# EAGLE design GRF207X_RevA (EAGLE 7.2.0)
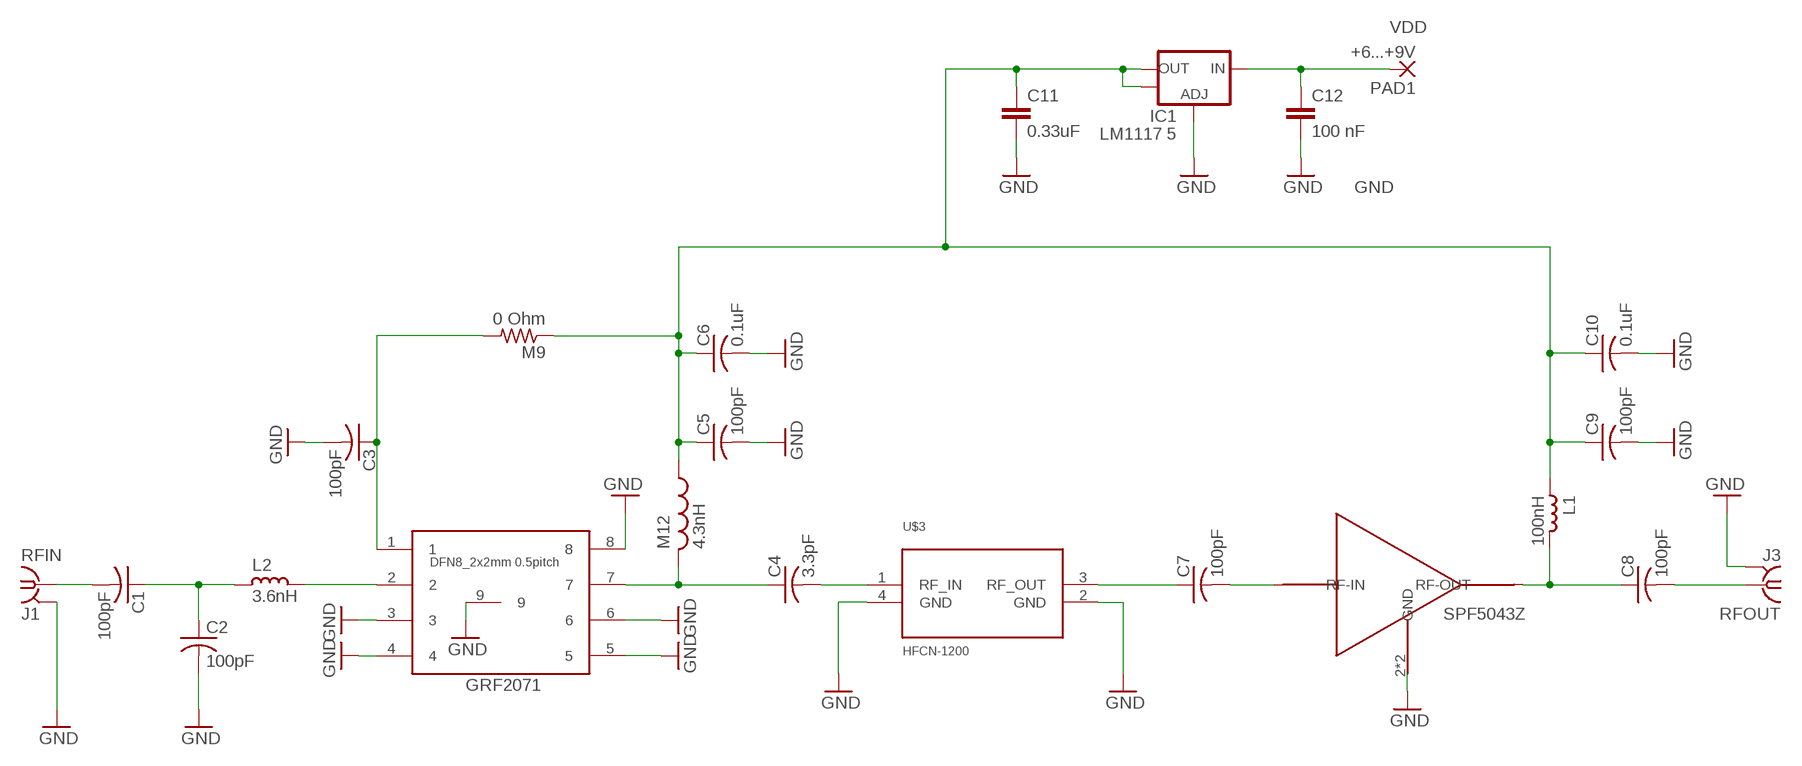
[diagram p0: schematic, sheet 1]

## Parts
C1  100pF  RCL_C0402_GRF30WIDE  [RCL_C-US_GRF_30WIDE]
C2  100pF  RCL_C0402_GRF30WIDE  [RCL_C-US_GRF_30WIDE]
C3  100pF  RCL_C0402_GRFWIDE  [RCL_C-US_GRF_NARROW]
C4  3.3pF  RCL_C0402_GRF30WIDE  [RCL_C-US_GRF_30WIDE]
C5  100pF  C-USC0603  [C0603]
C6  0.1uF  RCL_C0402_GRF30WIDE  [RCL_C-US_GRF_30WIDE]
C7  100pF  C-USC0603  [C0603]
C8  100pF  C-USC0603  [C0603]
C9  100pF  C-USC0603  [C0603]
C10  0.1uF  C-USC0603  [C0603]
C11  0.33uF  C-EUC0805  [C0805]
C12  100 nF  C-EUC0805  [C0805]
IC1  LM1117 5  V_REG_LM1117SOT223  [SOT223]
L1  100nH  L_0603  [L0603]
L2  3.6nH  L_0603  [L0603]
M9  0 Ohm  R-US_R0402  [R0402]
M12  4.3nH  L-US_L0402_WIDENORMAL  [RCL_L-US_L0402]
PAD1  +6...+9V  WIREPAD1,6/0,8  [1,6/0,8]
RFIN  J1  SMA-142-0701-801/806  [J502-ND-142-0701-801/806]
RFOUT  J3  SMA-142-0701-801/806  [J502-ND-142-0701-801/806]
SPF5043Z  SPF5043Z  PSA4-5043+  [PSA4-5043+]
U1  DFN8_2X2MM  [DFN8_2X2MM]
U$3  HFCN-1200  [HFCN-1200]

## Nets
GND: C2.2 C3.2 C5.2 C6.2 C9.2 C10.2 C11.2 C12.2 IC1.1(ADJ) RFIN.G@1 RFIN.G@2 RFIN.G@3 RFIN.G@4 RFOUT.G@1 RFOUT.G@2 RFOUT.G@3 RFOUT.G@4 SPF5043Z.2(GND) SPF5043Z.4(GND) U1.3 U1.4 U1.5 U1.6 U1.8 U1.9 U$3.2(GND) U$3.4(GND)
N$1 [RFIN]: C1.2 RFIN.1
N$2 [POWER]: C5.1 C6.1 C9.1 C10.1 C11.1 IC1.2(OUT) IC1.4(OUT) L1.2 M9.1 M12.1
N$3 [RFOUT]: C4.2 U$3.1(RF_IN)
N$4 [RFIN]: L2.1 U1.2
N$5 [RFOUT]: C7.1 U$3.3(RF_OUT)
N$6 [RFIN]: C1.1 C2.1 L2.2
N$7 [RFOUT]: C4.1 M12.2 U1.7
N$8 [RFOUT]: C7.2 SPF5043Z.3(RF-IN)
N$9 [RFOUT]: C8.1 L1.1 SPF5043Z.1(RF-OUT)
N$10 [RFOUT]: C8.2 RFOUT.1
N$11 [POWER]: C12.1 IC1.3(IN) PAD1.1(P)
VRX [POWER]: C3.1 M9.2 U1.1

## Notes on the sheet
- VDD
- GND
- SPF5043Z
- GRF2071

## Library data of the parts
C1-C4 C6 = GuerrillaRF:RCL_C0402_GRF
C5 C7-C10 = adafruit:C-US: CAPACITOR, American symbol
C11 C12 = resistor:C-EU: CAPACITOR, European symbol
IC1 = SparkFun-PowerIC:V_REG_LM1117: Voltage Regulator LM1117 Standard adjustable voltage regulator but in SMD form. Spark Fun Electronics SKU : COM-00595
L1 L2 = rc-master-smd:L_: INDUCTOR
M9 = rcl:R-US_: RESISTOR, American symbol
M12 = GuerrillaRF:L-US_L0402_WIDE
PAD1 = wirepad:WIREPAD: Wire PAD connect wire on PCB
RFIN RFOUT = GuerrillaRF:SMA-: SMA 50 Ohm End Launch Jack Receptacle - Round Contact; MF: JOHNSON COMPONENTS; MPN: 142-0701-801; OC_FARNELL: 1608592; OC_NEWARK: 90F2624
SPF5043Z = Ava:PSA4-5043+
U1 = GuerrillaRF:DFN8_2X2MM
U$3 = HFCN-1200:HFCN-1200: HFCN-1200+ HFCN-1200 High Pass Filter

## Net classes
0 default: drill 0.152 mm, clearance 0.152 mm
1 RFIN: clearance 0.508 mm to class 0
2 RFOUT: clearance 0.508 mm to class 0
3 POWER: clearance 0.254 mm to class 0
4 FID: clearance 0.178 mm to class 0
5 NC: clearance 0.178 mm to class 0
6 Bypass: clearance 0.203 mm to class 0

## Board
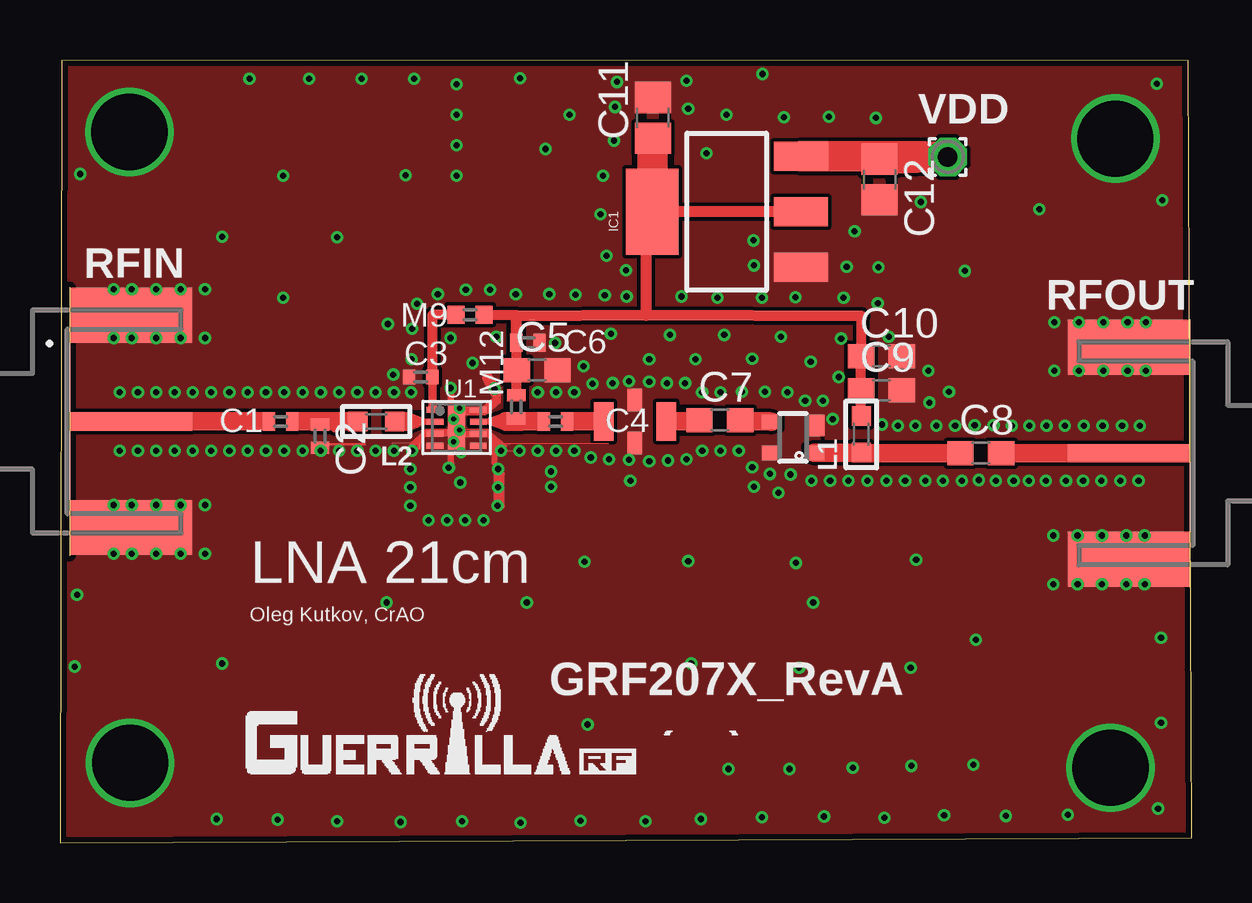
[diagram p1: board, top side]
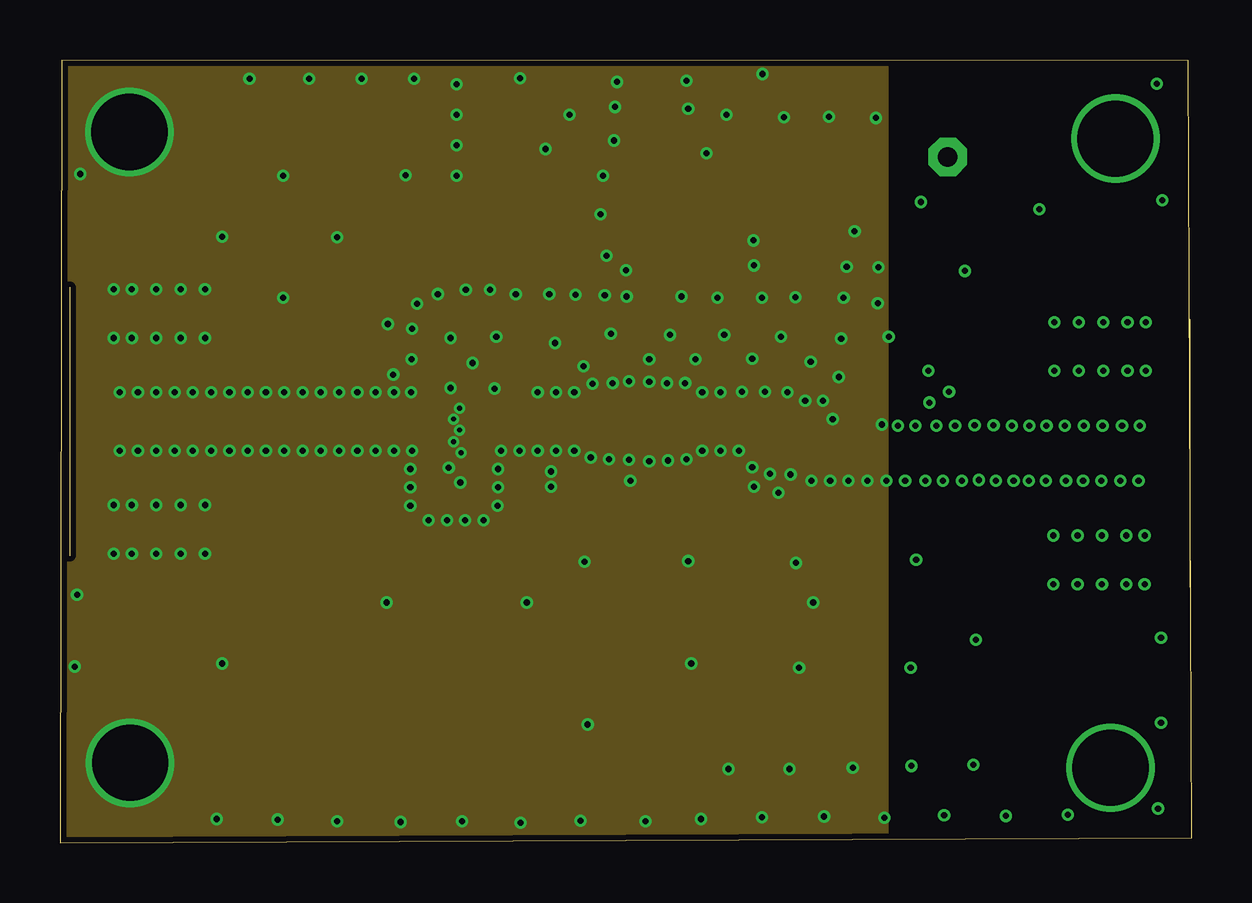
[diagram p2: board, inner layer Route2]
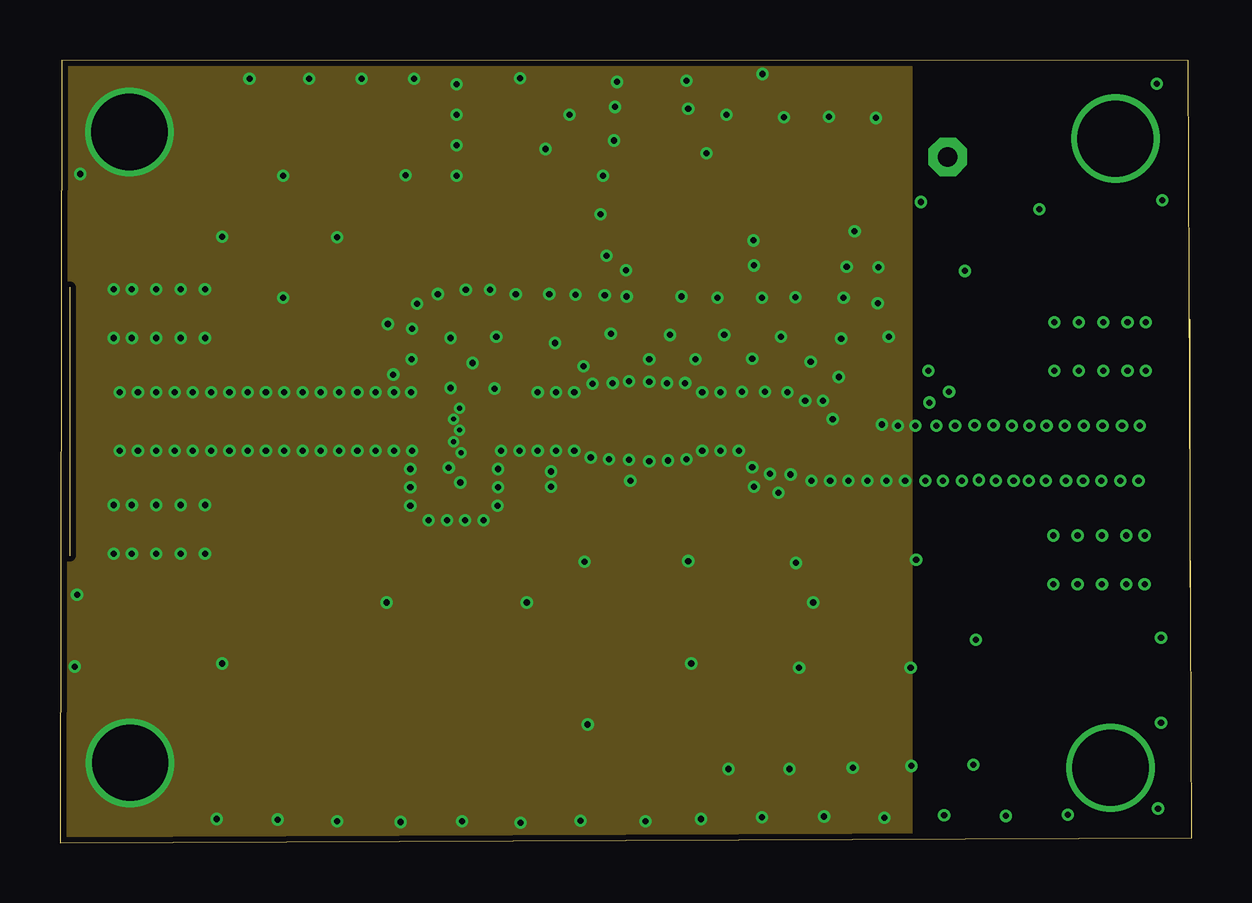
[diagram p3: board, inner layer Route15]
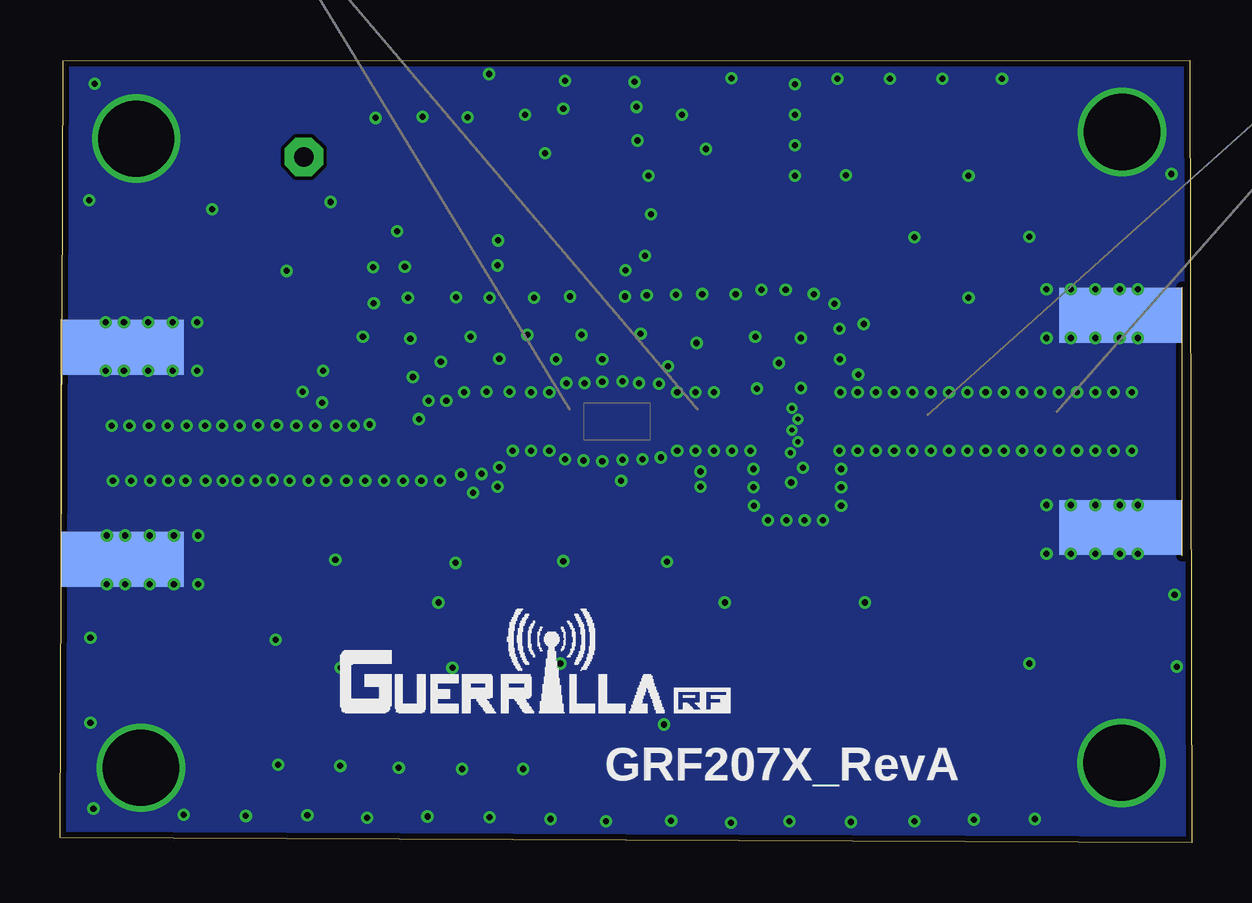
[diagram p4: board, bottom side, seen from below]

Size 47.17 x 32.61 mm. Coordinates in mm from the lower left corner, seen from the top.
Outline: 0,0 47.17,0.2 47.04,32.59 0.08,32.61 0,0
Copper layers (1*2*15*16): Top 0.035559375mm / dielectric 16mil / Route2 0.035559375mm / dielectric 24mil / Route15 0.035559375mm / dielectric 16mil / Bottom 0.035559375mm
Design rules "Eugene_Design_Rules_rev2": minimum track width 1mil, minimum drill 8mil, track to track 6mil, track to pad 4mil, pad to pad 4mil, via to via 4mil, smd to smd 0mil, copper to edge 10mil, drill to drill 8mil, minimum pad ring 5mil, minimum via ring 5mil, stop-mask expansion 0mil, vias tented up to drill 10mil, thermal gap 0mil

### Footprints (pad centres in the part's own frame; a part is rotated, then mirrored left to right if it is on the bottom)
RCL_C-US_GRF_30WIDE = smd 0.508 x 0.762: 1 -0.483,0; 2 0.483,0
RCL_C-US_GRF_NARROW = smd 0.508 x 0.61: 1 -0.483,0; 2 0.483,0
C0603 = smd 1.1 x 1: 1 -0.85,0; 2 0.85,0
C0805 = smd 1.3 x 1.5: 1 -0.85,0; 2 0.85,0
SOT223 = smd 1.219 x 2.235: 1 -2.311,-3.099; 2 0,-3.099; 3 2.311,-3.099 | smd 3.6 x 2.2: 4 0,3.099
L0603 = smd 0.8 x 0.8: 1 -0.762,0; 2 0.762,0
R0402 = smd 0.711 x 0.762: 1 -0.584,0; 2 0.584,0
RCL_L-US_L0402 = smd 0.508 x 0.762: 1 -0.483,0; 2 0.483,0
1,6/0,8 = drill 0.813 pad 1.6 octagon: 1 0,0
J502-ND-142-0701-801/806 = smd 5.08 x 0.762: 1 2.565,0 | smd 5.08 x 2.286: G@1 2.565,4.42; G@2 2.565,-4.42 | smd 5.08 x 2.286 bottom: G@3 2.565,4.42; G@4 2.565,-4.42
PSA4-5043+ = smd 0.6 x 0.8: 1 -0.65,-0.9; 3 0.65,0.9; 4 -0.65,0.9 | smd 0.9 x 0.8: 2 0.5,-0.9
DFN8_2X2MM = smd 0.7 x 0.25: 1 -0.9,0.75; 2 -0.9,0.25; 3 -0.9,-0.25; 4 -0.9,-0.75; 5 0.9,-0.75; 6 0.9,-0.25; 7 0.9,0.25; 8 0.9,0.75 | smd 0.7 x 1.8: 9 0,0
HFCN-1200 = smd 0.813 x 1.6: 1 -0.406,0; 3 2.21,0 | smd 0.61 x 0.94: 2 0.889,-0.889; 4 0.889,0.889

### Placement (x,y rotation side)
C1  9.19,17.55 180 top
C2  10.85,16.94 270 top
C3  15.04,19.41 180 top
C4  20.65,17.55 0 top
C5  19.89,19.69 0 top
C6  19.51,20.83 0 top
C7  27.51,17.6 0 top
C8  38.38,16.23 0 top
C9  34.24,18.85 0 top
C10  34.24,20.27 0 top
C11  24.71,30.2 90 top
C12  34.16,27.64 270 top
IC1  27.79,26.29 90 top
L1  33.4,17.02 90 top
L2  13.18,17.55 180 top
M9  17.09,22 180 top
M12  19.02,18.16 270 top
PAD1  37.01,28.58 0 top
RFIN  0.41,17.55 0 top
RFOUT  47.12,16.23 180 top
SPF5043Z  30.56,16.89 90 top
U1  16.54,17.3 0 top
U$3  23.06,17.55 0 top

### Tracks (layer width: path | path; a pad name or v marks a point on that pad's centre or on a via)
GND  (via drill 0.2, 0.25, 3.17)
  Top 0.051: 14.61,16.64 15.27,17.22 16.28,17.22 | 14.61,16.64 13.84,16.64 v13.92,16.33 | 14.61,16.64 14.73,16.64 14.66,16.51 | 15.44,17.07 15.65,17.04 | 15.65,17.04 16.54,16.92 v16.66,17.2 | 11,16.61 11.63,16.61 v11.63,16.33 | 21.44,16.64 22.86,16.64 | v21.44,16.33 21.44,16.64 | 18.21,15.6 18.16,15.6 18.26,15.39 | U1.3 15.65,17.04 | v16.21,15.62 16.31,15.8 | 14.99,16.41 14.73,16.38 v14.68,16.33 | 18.34,18.34 17.73,17.83 16.89,17.83 v16.66,18.11 | 18.36,18.95 18.34,18.34 | 16.87,17.22 17.81,17.22 18.49,16.64 18.82,16.64 | 18.82,16.64 21.44,16.64 | 16.89,16.92 17.83,16.92 | 17.83,16.92 18.52,16.33 19.41,16.33 | 17.68,18.01 U1.8 | 17.81,17.07 U1.6 | 17.83,17.04 U1.6 | 17.83,16.92 U1.6 | 18.49,16.51 18.82,16.64 | 18.11,15.85 v18.26,15.57 | 18.34,18.34 17.92,18.22 | 15.01,16.84 14.95,16.57
  Top 0.102: 11,16.61 12.7,16.61 | 15.01,16.84 14.99,16.41 | 15.09,16.87 14.95,16.57 14.88,16.43
  Top 0.254: 14.66,16.51 15.29,17.09 16.26,17.09 | 15.44,17.07 16.46,17.07 | 18.21,14.25 18.21,15.6 | 18.42,14.02 18.42,15.37 | 16.31,15.8 16.31,17.15 | 16.87,17.07 17.81,17.07 | 18.49,16.51 17.83,17.04 | 18.11,15.85 18.11,16.79 | 16.31,17.32 16.31,18.67
  Top 0.356: 16.87,18.01 17.68,18.01 | 17.68,18.01 17.7,18.01 | 17.68,18.01 17.92,18.22 18.19,18.44
  Top 0.457: 17.83,19.35 18.16,18.75
  other vias: 31.06,18.42 31.8,18.42 34.93,17.37 35.66,17.37 27.53,18.77 26.77,18.77 26.06,19.15 25.3,19.15 24.56,19.2 23.72,19.23 21.44,18.77 20.68,18.77 30.45,15.34 28.85,15.65 29.59,15.37 28.3,16.33 27.53,16.33 26.77,16.33 26.11,15.98 25.35,15.93 24.56,15.9 23.72,15.95 22.89,15.98 22.12,16.05 20.68,16.33 41.45,19.66 42.47,19.66 43.48,19.66 44.5,19.66 41.45,21.69 42.47,21.69 43.48,21.69 44.5,21.69 41.4,12.8 42.42,12.8 41.4,10.77 42.42,10.77 43.43,10.77 43.43,12.8 44.45,10.77 44.45,12.8 45.21,12.8 45.21,10.77 45.26,19.66 45.26,21.69 2.92,3.33 2.9,29.62 43.99,29.34 23.04,19.15 22.2,19.13 9.35,18.77 8.59,18.77 7.82,18.77 7.06,18.77 6.3,18.77 5.54,18.77 4.78,18.77 4.01,18.77 3.25,18.77 2.49,18.77 2.49,16.33 3.25,16.33 4.01,16.33 4.78,16.33 5.54,16.33 6.3,16.33 7.06,16.33 7.82,16.33 8.59,16.33 9.35,16.33 6.05,14.07 5.03,14.07 4.01,14.07 3,14.07 3,12.04 4.01,12.04 5.03,12.04 6.05,12.04 5.03,23.06 4.01,23.06 3,23.06 6.05,21.03 5.03,21.03 4.01,21.03 3,21.03 2.24,14.07 2.24,12.04 2.24,21.03 6.05,23.06 2.24,23.06 19.91,16.33 6.76,7.47 6.76,25.25 16.54,30.33 16.54,27.79 16.54,31.6 16.54,29.06 10.11,18.77 10.11,16.33 43.79,3.12 22,4.93 19.46,10.01 13.61,10.01 31.39,10.01 26.31,7.47 21.23,30.33 20.4,22.86 20.24,28.91 9.3,22.71 10.87,18.77 11.63,18.77 12.4,18.77 13.16,18.77 13.92,18.77 13.16,16.33 10.87,16.33 12.4,16.33 19.15,16.33 19.91,18.77 9.3,27.79 14.63,18.77 16.28,21.03 18.19,21.08 16.41,17.65 16.41,16.71 16.28,18.95 16.71,16.26 13.89,19.51 14.66,20.14 21.82,19.85 20.63,20.82 19,22.85 23.77,15.09 14.61,14.05 20.47,15.47 20.47,14.83 14.61,14.81 14.61,15.57 18.26,14.81 18.24,14.05 16.69,15.01 18.39,16.33 15.37,13.44 16.13,13.44 16.89,13.44 17.65,13.44 17.2,19.99 18.11,18.92 28.42,18.8 29.39,18.8 30.33,18.77 28.93,14.83 32.21,17.65 32.46,19.41 32.56,21.01 30.05,21.08 31.29,20.04 27.69,21.16 25.43,21.16 22.96,21.21 28.85,20.17 26.49,20.14 24.56,20.14 34.26,17.42 31.32,15.09 29.95,14.58 32.11,15.09 32.87,15.09 36.53,17.37 37.31,17.37 38.13,17.4 38.91,17.4 39.67,17.37 40.41,17.37 41.12,17.37 41.88,17.37 42.67,17.37 43.46,17.37 44.27,17.37 45.01,17.37 33.66,15.09 34.44,15.09 35.23,15.09 36.07,15.09 36.8,15.09 37.59,15.09 38.3,15.11 39.01,15.09 39.75,15.09 40.39,15.09 41.1,15.09 41.94,15.09 42.65,15.09 43.41,15.09 44.2,15.09 44.96,15.09 22.63,27.79 22.53,26.19 21.49,22.83 22.71,22.81 23.62,22.76 23.6,23.85 22.78,24.46 23.09,29.26 23.14,30.66 23.22,31.7 26.11,31.75 26.19,30.58 26.95,28.73 35.89,26.7 30.66,22.73 32.66,22.71 34.09,22.48 34.54,21.08 36.2,19.66 37.06,18.8 36.25,18.34 25.91,22.76 27.41,22.71 29.26,22.71 7.9,31.83 0.84,27.86 45.72,31.62 37.72,23.83 40.82,26.39 45.95,26.77 30.81,7.29 35.46,7.29 26.72,0.99 31.85,1.09 36.86,1.14 45.77,1.42 45.9,5 45.9,8.53 26.19,11.73 35.69,11.79 6.53,0.99 0.61,7.34 30.18,30.23 32.05,30.25 34.01,30.2 27.79,30.33 33.12,25.48 11.56,25.22 14.4,27.81 14.88,22.45 14.68,21.41 15.75,22.86 17.93,23.04 16.92,23.04 9.07,0.97 11.56,0.89 14.2,0.86 16.76,0.89 19.2,0.84 21.69,0.91 24.41,0.89 0.71,10.34 10.39,31.83 12.57,31.83 14.76,31.83 19.18,31.85 29.29,32.03 29.26,1.07 34.37,1.04 39.42,1.12 42.01,1.17 35.48,3.2 33.05,3.12 30.4,3.07 27.86,3.07 38.07,3.25 38.18,8.46 30.68,11.66 21.87,11.71 13.67,21.62 32.79,24 28.93,24.05 28.91,25.1 34.11,23.98
  pour Bottom: 0.25,33.45 47.22,33.4 47.02,0.53 0.33,0.18
  pour Top: 0.03,33.55 47.19,33.66 47.19,0.38 0.03,0.28
  pour Route2: -0.48,34.06 34.32,34.06 34.32,-0.74 -0.48,-0.74
  pour Route15: -0.99,34.82 35.33,34.82 35.33,-1.75 -0.99,-1.75
  pour Top: 30.48,18.16 30.48,17.25 30.45,17.22 29.9,16.66 29.85,16.66 29.69,16.51 29.69,15.88 29.82,15.75 30.56,15.75 30.58,15.77 30.58,16.38 30.56,16.41 31.12,16.97 31.12,18.01 31.22,18.11 30.71,18.11 30.66,18.16
N$1
  Top 0.254: C1.2 8.53,17.55
  Top 0.762: 8.53,17.55 RFIN.1
N$2
  Top 0.356: 19.02,22 19.02,21.87
  Top 0.406: M9.1 19.02,22 | C9.1 33.35,18.47 | L1.2 33.39,17.78 33.39,18.57 | 33.35,18.57 33.39,18.57 | 33.39,18.57 33.39,18.75 | 33.43,18.75 33.39,18.75 | C9.1 C10.1 33.4,20.27 33.4,21.95 | 33.39,18.75 C9.1 | M12.1 19.04,18.64 C5.1 19.02,19.69 C6.1
  Top 0.457: C6.1 19.02,21.87 19.02,21.95 24.43,21.97 | 33.4,21.95 24.43,21.97 | IC1.2 IC1.4 24.43,26.59 24.43,21.97
  Top 1.27: C11.1 24.69,29.35 IC1.4
N$3
  Top 0.254: C4.2 21.26,17.55
  Top 0.762: 21.26,17.55 U$3.1
N$4
  Top 0.051: U1.2 15.64,17.48 15.34,17.48 14.58,17.2 14,17.2 | U1.2 15.64,17.63 15.34,17.63 14.58,17.91 14.05,17.91 | 15.04,17.45 15.58,17.45 15.58,17.55 U1.2 | 15.6,17.55
  Top 0.203: 15.06,17.55 15.6,17.55
  Top 0.229: U1.2 15.6,17.55
  Top 0.356: 14.83,17.55 15.06,17.55
  Top 0.406: L2.1 14.05,17.55
  Top 0.508: 14.55,17.55 14.83,17.55
  Top 0.711: 14.45,17.55 14.55,17.55
  Top 0.762: 14.05,17.55 14.45,17.55
N$5
  Top 0.406: 26.8,17.55 25.73,17.55 25.73,17.6 25.48,17.6 25.48,17.58 | 25.48,17.58 25.32,17.58 | 25.48,17.58 26.66,17.58 C7.1
  Top 0.762: 26.8,17.55 U$3.3
N$6
  Top 0.254: C1.1 9.83,17.55
  Top 0.406: C2.1 11.46,17.42 | 11.46,17.42 11.46,17.3 | 11.46,17.42 11.46,17.55
  Top 0.762: L2.2 11.46,17.55 9.83,17.55
N$7
  Top 0.051: 19.28,17.2 18.49,17.2 17.73,17.48 U1.7 | 19.2,17.91 18.49,17.91 17.73,17.63 U1.7 | 17.96,17.55 17.89,17.45 17.71,17.45 U1.7
  Top 0.254: 18.72,17.55 18.85,17.68 M12.2
  Top 0.305: 17.91,17.55 17.96,17.55 18.36,17.55
  Top 0.457: 20.04,17.55 C4.1
  Top 0.508: 18.21,17.55 18.36,17.55 18.72,17.55
  Top 0.762: 20.04,17.55 18.72,17.55 18.57,17.55
N$8
  Top 0.406: 28.42,17.55 29.54,17.55 29.54,17.53 28.36,17.53 C7.2
  Top 0.762: 28.42,17.55 29.55,17.55 SPF5043Z.3
N$9
  Top 0.406: L1.1 33.35,16.26 33.35,16.24 33.35,16.23
  Top 0.762: SPF5043Z.1 33.35,16.24 | 37.69,16.23 C8.1 33.35,16.23
N$10
  Top 0.254: 39.09,16.26 39.09,16.23
  Top 0.406: 39.09,16.26 39.23,16.26 C8.2
  Top 0.762: 39.09,16.23 C8.2 RFOUT.1 44.91,16.23
N$11
  Top 1.27: PAD1.1 36.8,28.58 | 35.99,28.6 C12.1 36.8,28.58 | IC1.3 35.99,28.6 | 35.99,28.6 36.8,28.58
VRX
  Top 0.254: U1.1 15.53,18.16
  Top 0.356: 15.53,18.14 15.53,18.16 15.53,19.35 C3.1
  Top 0.406: C3.1 15.52,22 16.33,22 M9.2

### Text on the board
Route2: Metal Layer 2 Ground Plane
Route15: Metal Layer 3 Ground Plane
Bottom: Bottom Copper
tNames: VDD | LNA 21cm | Oleg Kutkov, CrAO | GRF207X_RevA
bNames: GRF207X_RevA
tStop: Top Soldermask
bStop: Bottom Soldermask
tCream: Solder Paste Top
bCream: Solder Paste Bottom
Drills: Drill Drawing
bDocu: REV | Description | Date | 1 | Initial release | 05/04/2017 | Required files: / See Readme | Note A: | Note A: | Specifications: / All units are in inches unless otherwise specified. / 1. Materials / Beginning foil thickness 1/2oz min. but shall meet the minimum requirements below: / Layer 1 - Top Layer, 1 oz copper, 0.0014 / Dielectric - Rogers 4003, 0.016 +/- 0.0006 / Layer 2 - Ground Plane, 1 oz copper, 0.0014 / Dielectric - Fr4, (adjust this layer to meet thickness target) / Layer 3 - Ground Plane, 1 oz copper, 0.0014 / Dielectric - Rogers 4003, 0.016 +/- 0.0006 / Layer 4 - Bottom Layer, 1 oz copper, 0.0014 / / Total Board Thickness = 0.062 +/- 0.005 including top and bottom soldermask. / / 2. Hole Plating / Copper plate 0.0010/0.0015 thick in Thru Hole Vias (Approx. 0.0015 on surface). / / 3. Finish / ENIG / Thickness 3-8 micro inches. / Solder Mask / Liquid Photo Imagable (LPI) Solder Mask Over Bare Copper (SMOBC) on Both Sides of PCB. / Color: Red or Approved Equal. / Silkscreen: White Non-Conductive Epoxy Ink. / Supplier ID and Lot Number shall be noted on bottom silkscreen. / 4. Tolerances / Overall board dimension tolerance +/- 0.010. / Hole Diameter >= 0.100 +/- 0.005. / Hole Diameter < 0.100 +/- 0.003. / Layer to layer registration should be +/- 0.001. / All holes shall be located within hole to pad tangency. / 5. Traces / Conductors indicated as Note A shall be 0.030 +/- 0.001 wide and have a coplanar / ground spacing of 0.020 +/- 0.001 Manufacturer shall test for lines indicated to be / 50 Ohm +/- 10% and may adjust the width as needed. / Minimum conductor width is 0.006 +/- 0.001. / Minimum conductor to conductor spacing is 0.006. / TDR coupon required to be delivered with boards. / The controlled impedance on layer 1 shall be 50 Ohms +/- 10%. | SIZE | DOCUMENT NO. | REV | Dimensions are in inches unless / otherwise specified. | A | GRF207X | Date: | Drawn By: Eugenio M. Proenza | SCALE NONE | Sheet 1 of 1 | 05/04/2017
DrillLegend: LAYER-STACK
DrillLegend_01-16: 01-16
